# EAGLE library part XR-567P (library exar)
TONE DECODER
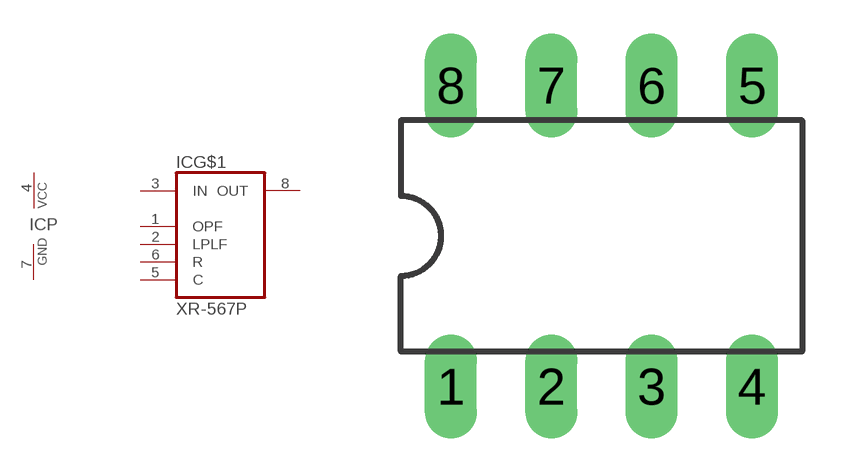
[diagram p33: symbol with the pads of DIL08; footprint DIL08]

Designator prefix IC; gates G$1=XR-567 P=PWRN

## XR-567P (OC_FARNELL: unknown; OC_NEWARK: unknown)  [DIL08]
1  G$1:OPF  in
2  G$1:LPLF  in
3  G$1:IN  in
4  P:VCC  pwr
5  G$1:C  in
6  G$1:R  in
7  P:GND  pwr
8  G$1:OUT  out

## Footprint DIL08 (pad centres in mm)
Dual In Line Package
drill 0.813 long: 1 -3.81,-3.81; 2 -1.27,-3.81; 3 1.27,-3.81; 4 3.81,-3.81; 5 3.81,3.81; 6 1.27,3.81; 7 -1.27,3.81; 8 -3.81,3.81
